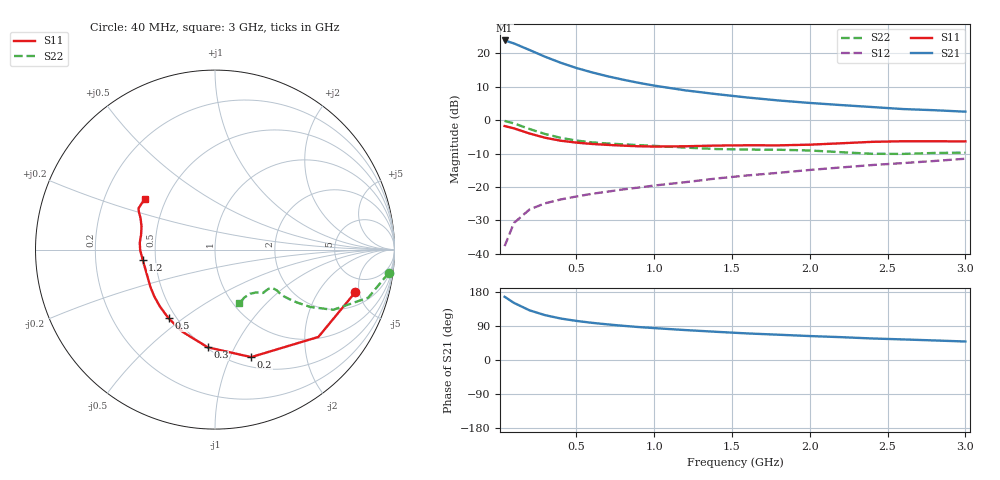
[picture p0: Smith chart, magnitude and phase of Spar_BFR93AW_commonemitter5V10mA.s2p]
! Filename:  BFR93AWB.S2P  Version:  4.0
! NXP part #: BFR93AW  Date: Jun 1994
! Bias condition: Vce=5V, Ic=10mA
#  MHz  S  MA  R  50
! Freq  S11  S21  S12  S22  !GUM [dB]
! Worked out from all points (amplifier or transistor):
!   21 points, 40 MHz to 3 GHz, reference 50 ohm
!   highest |S21| = 23.9 dB at 40 MHz (marker M1)
!   |S21| within 3 dB of that: start of sweep to 207.1 MHz
!   unconditionally stable (mu >= 1): 949.9 MHz to end of sweep
!   at 300 MHz: K = 0.52, MSG = 21.9 dB, |S12| = -24.9 dB
!   at 1 GHz: K = 1.02, MAG = 14.1 dB, |S12| = -19.6 dB
!   at 3 GHz: K = 1.03, MAG = 6.0 dB, |S12| = -11.5 dB
!   lowest NFmin = 1.40 dB at 500 MHz
!   S11 on the Smith chart (normalised r, x): 40 MHz: 3.20, -4.56; 200 MHz: 0.60, -1.20; 300 MHz: 0.51, -0.79; 500 MHz: 0.45, -0.44; 1.2 GHz: 0.42, -0.06; 3 GHz: 0.38, +0.28
40  0.817 -16.9  15.62 166.9  0.013 81.0  0.976 -7.7
100  0.754 -40.2  14.11 150.7  0.029 70.1  0.895 -17.4
200  0.632 -71.4  11.24 131.1  0.046 59.4  0.739 -27.0
300  0.546 -94.2  8.916 118.3  0.057 54.4  0.621 -31.0
400  0.493 -111.4  7.247 109.5  0.065 53.4  0.545 -32.8
500  0.462 -124.0  6.06 103.2  0.072 53.6  0.496 -33.7
600  0.441 -134.3  5.208 98.2  0.079 55.3  0.466 -34.1
700  0.427 -142.5  4.552 94.0  0.085 56.7  0.448 -34.1
800  0.416 -149.8  4.044 90.3  0.092 58.2  0.435 -34.0
900  0.407 -156.2  3.631 87.0  0.098 59.8  0.424 -33.7
1000  0.403 -162.1  3.297 84.2  0.105 61.3  0.413 -33.4
1200  0.407 -172.2  2.798 79.0  0.118 63.8  0.389 -33.7
1400  0.417 -179.7  2.458 74.4  0.134 65.9  0.37 -36.1
1600  0.421 174.7  2.185 70.1  0.149 67.3  0.363 -39.8
1800  0.42 168.8  1.974 66.7  0.163 69.0  0.361 -42.0
2000  0.43 162.2  1.813 63.2  0.18 70.2  0.352 -43.3
2200  0.451 157.0  1.685 60.3  0.196 71.2  0.332 -45.9
2400  0.474 153.5  1.574 56.8  0.213 71.8  0.314 -51.6
2600  0.484 151.7  1.468 54.3  0.228 72.0  0.313 -58.6
2800  0.483 148.5  1.411 51.6  0.245 72.7  0.323 -63.1
3000  0.482 144.1  1.341 48.8  0.265 72.8  0.327 -65.8
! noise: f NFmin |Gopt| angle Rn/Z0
500  1.4  0.137  88.2  0.172
1000  1.9  0.24  145.7  0.198
2000  2.9  0.61  -152.3  0.131
